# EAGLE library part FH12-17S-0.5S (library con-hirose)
0.5mm Pitch Connectors For FPC/FFC Source: Data sheet
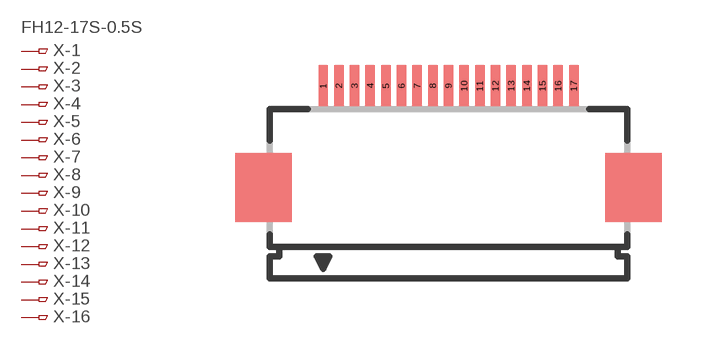
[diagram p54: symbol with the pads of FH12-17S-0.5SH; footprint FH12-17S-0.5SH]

Designator prefix X; gates -1=PINV -2=PIN -3=PIN -4=PIN -5=PIN -6=PIN -7=PIN -8=PIN -9=PIN -10=PIN -11=PIN -12=PIN -13=PIN -14=PIN -15=PIN -16=PIN -17=PIN

## FH12-17S-0.5SH (OC_FARNELL: unknown; OC_NEWARK: unknown)  [FH12-17S-0.5SH]
1  -1:1  pas
2  -2:1  pas
3  -3:1  pas
4  -4:1  pas
5  -5:1  pas
6  -6:1  pas
7  -7:1  pas
8  -8:1  pas
9  -9:1  pas
10  -10:1  pas
11  -11:1  pas
12  -12:1  pas
13  -13:1  pas
14  -14:1  pas
15  -15:1  pas
16  -16:1  pas
17  -17:1  pas

## Footprint FH12-17S-0.5SH (pad centres in mm)
0.5mm Pitch Connectors For FPC/FFC Source: Data sheet
smd 0.3 x 1.3: 1 -4,3.25; 2 -3.5,3.25; 3 -3,3.25; 4 -2.5,3.25; 5 -2,3.25; 6 -1.5,3.25; 7 -1,3.25; 8 -0.5,3.25; 9 0,3.25; 10 0.5,3.25; 11 1,3.25; 12 1.5,3.25; 13 2,3.25; 14 2.5,3.25; 15 3,3.25; 16 3.5,3.25; 17 4,3.25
